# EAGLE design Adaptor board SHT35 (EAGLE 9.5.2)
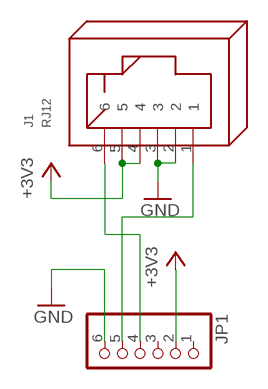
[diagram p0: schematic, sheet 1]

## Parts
J1  RJ12  [RJ12]
JP1  PINHD-1X6  [1X06]

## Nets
+3V3: J1.4 J1.5 JP1.2
GND: J1.2 J1.3 JP1.6
SCL: J1.6 JP1.4
SDA: J1.1 JP1.5
Unconnected: JP1.1 JP1.3

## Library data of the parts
J1 = con-rj:RJ12: RJ12, RJ14 and RJ25 RJ12, RJ14 and RJ25 jacks side mounted http://www.tycoelectronics.com
JP1 = pinhead:PINHD-1X6: PIN HEADER

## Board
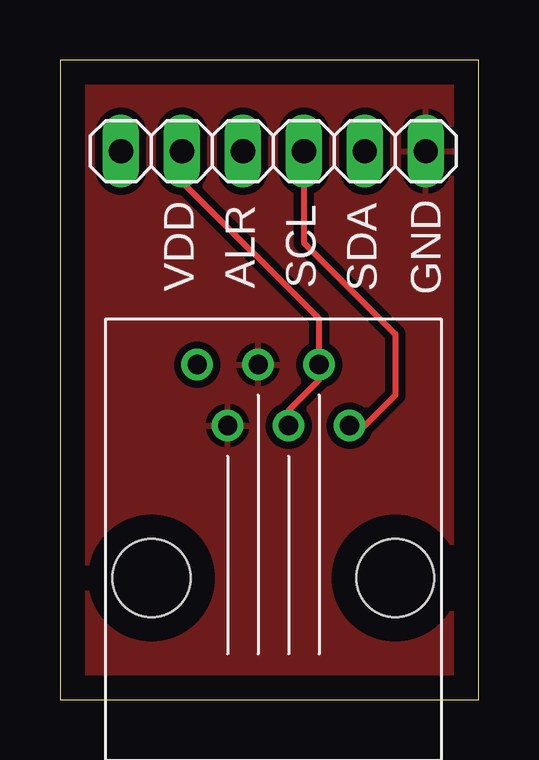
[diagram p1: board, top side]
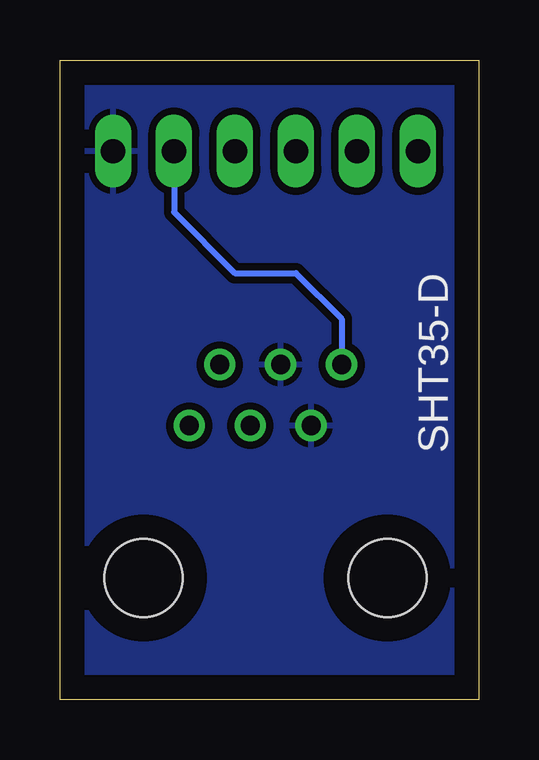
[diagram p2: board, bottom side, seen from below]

Size 17.45 x 26.66 mm. Coordinates in mm from the lower left corner, seen from the top.
Outline: 0,0 17.45,0 17.45,26.66 0,26.66 0,0
Copper layers (1*16): Top 0.035mm / dielectric 1.5mm / Bottom 0.035mm
Design rules "default": minimum track width 6mil, minimum drill 0.35mm, track to track 6mil, track to pad 6mil, pad to pad 6mil, via to via 6mil, smd to smd 6mil, copper to edge 40mil, drill to drill 6mil, minimum pad ring 10mil, minimum via ring 8mil, stop-mask expansion 4mil, vias tented up to drill 0mil, thermal gap 10mil

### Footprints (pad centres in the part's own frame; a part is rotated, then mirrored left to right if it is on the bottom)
RJ12 = drill 0.8: 1 -8.89,-3.175; 2 -6.35,-1.905; 3 -8.89,-0.635; 4 -6.35,0.635; 5 -8.89,1.905; 6 -6.35,3.175 | hole 3.25: 0,-5.08; 0,5.08
1X06 = drill 1.016 long: 1 -6.35,0; 2 -3.81,0; 3 -1.27,0; 4 1.27,0; 5 3.81,0; 6 6.35,0

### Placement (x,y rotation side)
J1  8.89,5.08 270 top
JP1  8.89,22.86 0 top

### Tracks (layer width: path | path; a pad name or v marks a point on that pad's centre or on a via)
+3V3
  Top 0.254: JP1.2 5.08,21.59 10.79,15.88 J1.5 10.79,13.34 9.52,12.06 J1.4
GND
  pour Bottom (isolate 0.305): 0,26.67 17.78,26.67 17.78,0 0,0
  pour Top (isolate 0.305): 0,26.67 17.78,26.67 17.78,0 0,0
SCL
  Top 0.254: JP1.4 10.16,19.05 13.97,15.24 13.97,12.7 12.7,11.43 J1.6
SDA
  Bottom 0.254: JP1.5 12.7,20.32 10.16,17.78 7.62,17.78 5.71,15.88 J1.1

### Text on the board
tPlace: VDD | ALR | SCL | SDA | GND
bPlace: SHT35-D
